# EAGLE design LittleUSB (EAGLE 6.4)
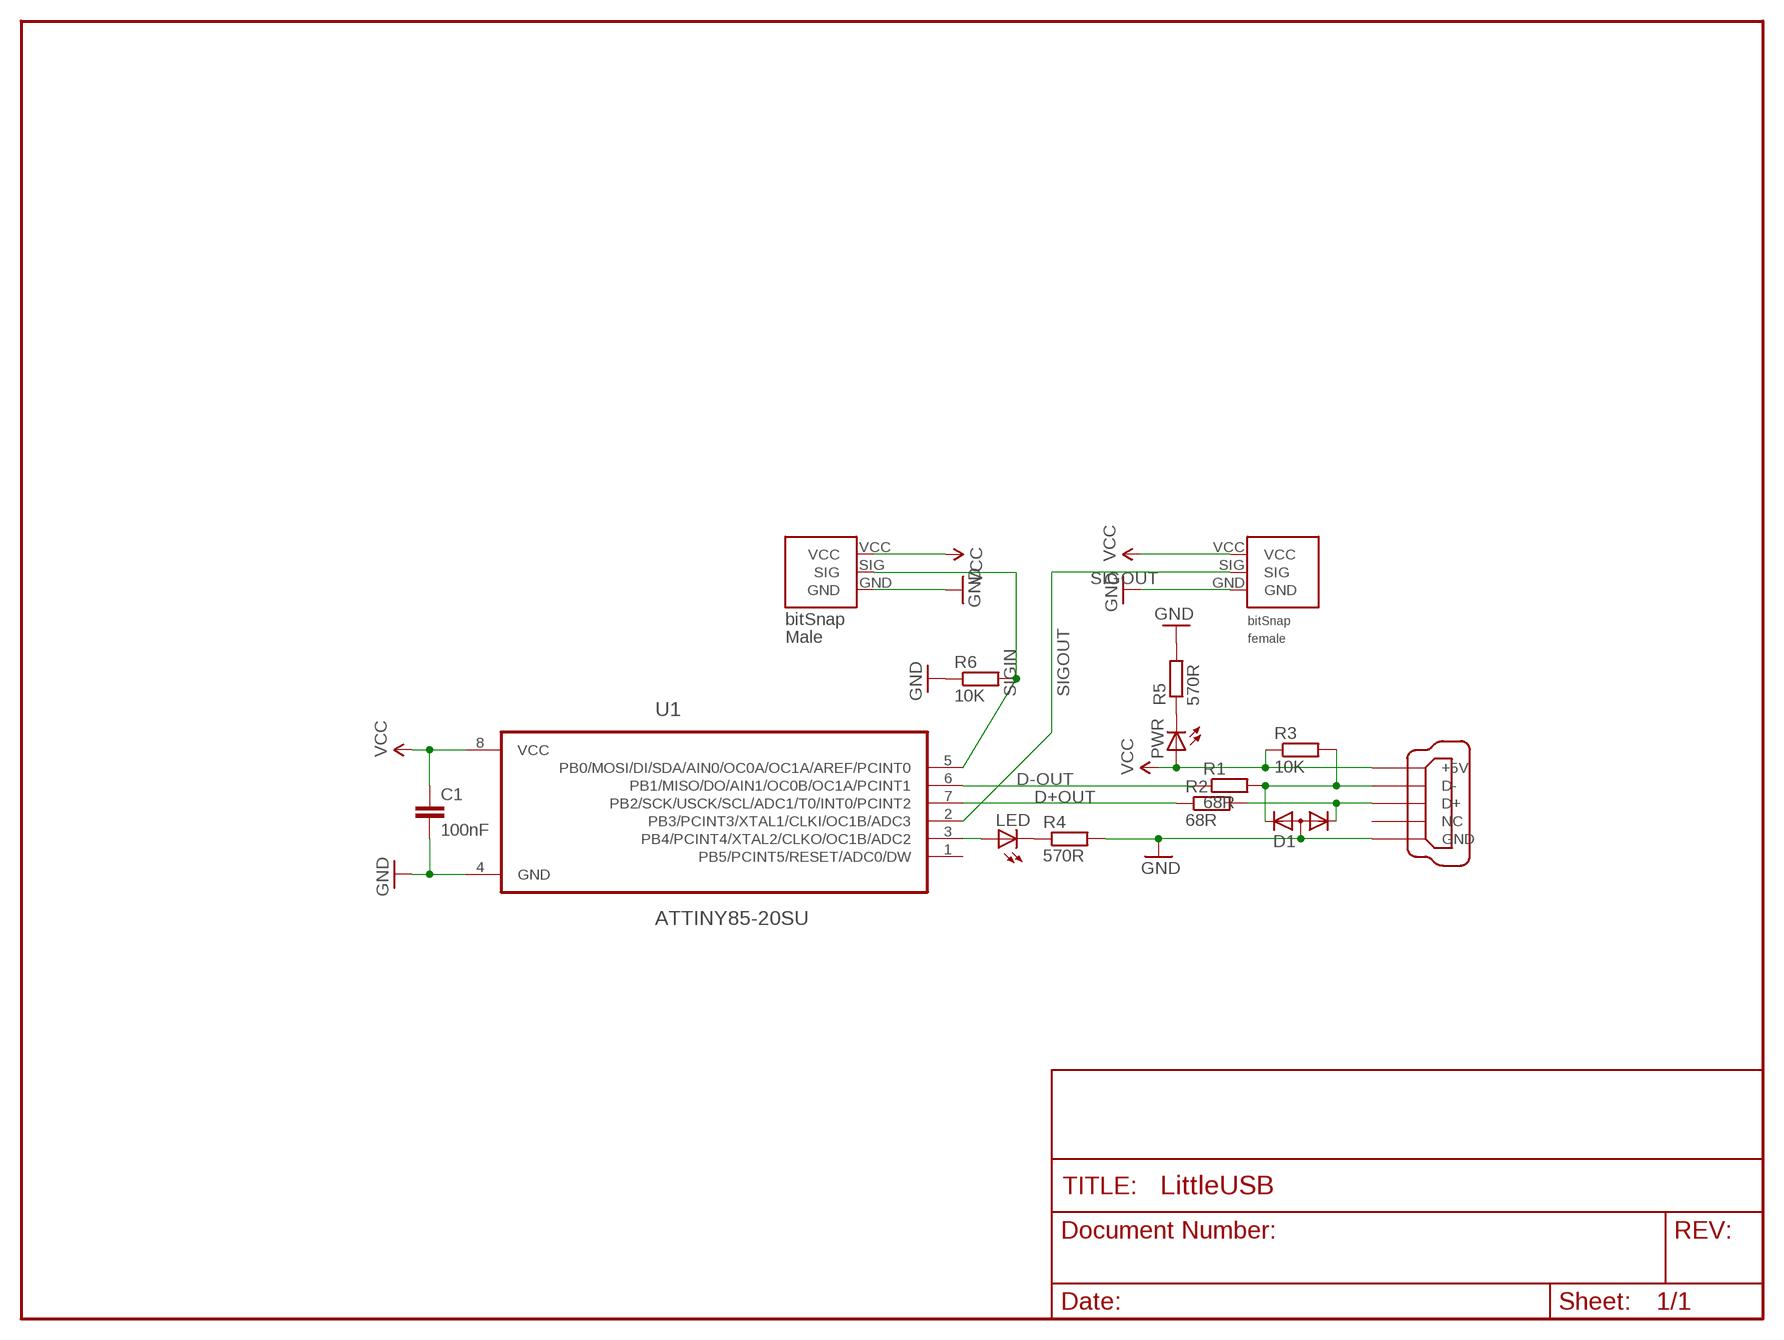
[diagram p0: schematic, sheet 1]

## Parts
C1  100nF  C-EUC0603  [C0603]
D1  DIODE-2CA|ACSOT23  [SOT23]
I3BSF  LITTLEBIT_FEMALE  [LITTLEBIT_FEMALE]
I3BSM  LITTLEBIT_MALE  [LITTLEBIT_MALE]
LED  LEDCHIPLED_0603  [CHIPLED_0603]
PWR  LEDCHIPLED_0603  [CHIPLED_0603]
R1  68R  R-EU_R0603  [R0603]
R2  68R  R-EU_R0603  [R0603]
R3  10K  R-EU_R0603  [R0603]
R4  570R  R-EU_R0603  [R0603]
R5  570R  R-EU_R0603  [R0603]
R6  10K  R-EU_R0603  [R0603]
U1  ATTINY85-20SU  [SOIC127P798X216-8N]
X1  MINI-USB-32005-301  [32005-301]

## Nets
D+OUT: R2.1 U1.7(PB2/SCK/USCK/SCL/ADC1/T0/INT0/PCINT2)
D-OUT: R1.1 U1.6(PB1/MISO/DO/AIN1/OC0B/OC1A/PCINT1)
GND: C1.2 D1.3(A) I3BSF.GND I3BSM.GND R4.2 R5.2 R6.1 U1.4(GND) X1.GND
N$1: LED.A U1.3(PB4/PCINT4/XTAL2/CLKO/OC1B/ADC2)
N$2: D1.2(K2) R1.2 R3.2 X1.D-
N$3: D1.1(K1) R2.2 X1.D+
N$4: LED.C R4.1
N$6: PWR.C R5.1
SIGIN: I3BSM.SIG R6.2 U1.5(PB0/MOSI/DI/SDA/AIN0/OC0A/OC1A/AREF/PCINT0)
SIGOUT: I3BSF.SIG U1.2(PB3/PCINT3/XTAL1/CLKI/OC1B/ADC3)
VCC: C1.1 I3BSF.VCC I3BSM.VCC PWR.A R3.1 U1.8(VCC) X1.+5V
Unconnected: U1.1(PB5/PCINT5/RESET/ADC0/DW) X1.NC

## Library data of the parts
C1 = rcl:C-EU: CAPACITOR, European symbol
D1 = diode:DIODE-2CA|AC: Dual DIODE Cathode-Anode|Anode-Cathode
I3BSF = MikesParts:LITTLEBIT_FEMALE
I3BSM = MikesParts:LITTLEBIT_MALE
LED PWR = led:LED: LED
R1-R6 = rcl:R-EU_: RESISTOR, European symbol
U1 = MikesParts:ATTINY85-20SU: 8-bit Microcontroller with In-System Programmable Flash; MPN: ATTINY85-20SU; OC_FARNELL: 1455164; OC_NEWARK: 58M3797; PACKAGE: SOIC-8; SUPPLIER: Atmel
X1 = MikesParts:MINI-USB-: MINI USB-B Conector Source: www.cypressindustries.com; OC_FARNELL: unknown; OC_NEWARK: unknown

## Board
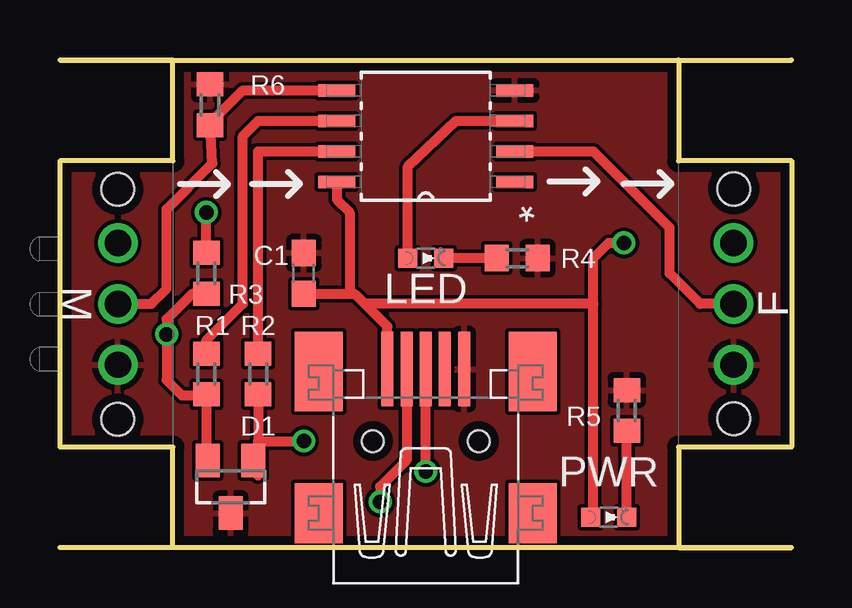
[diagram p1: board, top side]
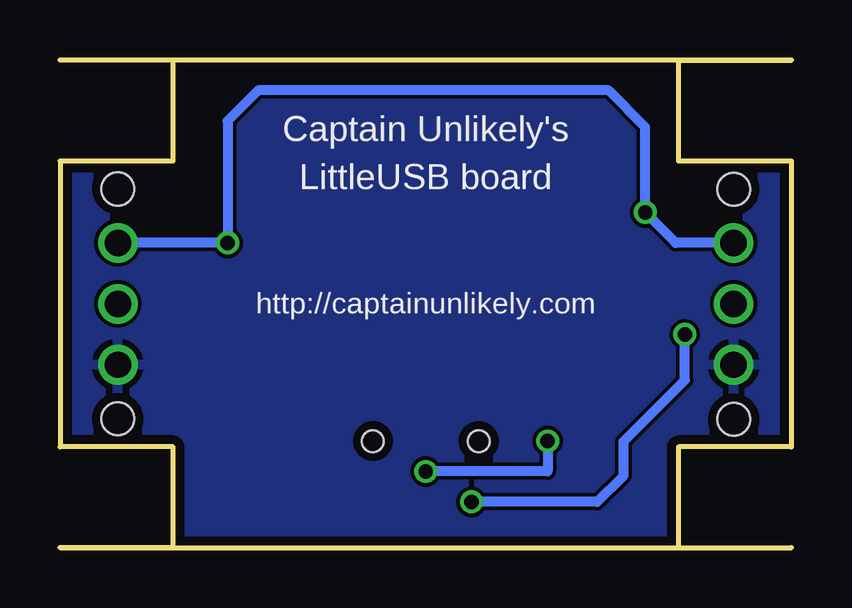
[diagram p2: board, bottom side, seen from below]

Size 30.48 x 20.32 mm. Coordinates in mm from the lower left corner, seen from the top.
Outline: 0,20.32 30.48,20.32
Outline: 30.48,0 0,0
Copper layers (1*16): Top 0.0356mm / dielectric 1.5011mm / Bottom 0.0356mm
Design rules "LaenPCBOrder": minimum track width 6mil, minimum drill 13mil, track to track 6mil, track to pad 6mil, pad to pad 6mil, via to via 6mil, smd to smd 6mil, copper to edge 15mil, drill to drill 6mil, minimum pad ring 7mil, minimum via ring 7mil, stop-mask expansion 4mil, vias tented up to drill 0mil, thermal gap 10mil

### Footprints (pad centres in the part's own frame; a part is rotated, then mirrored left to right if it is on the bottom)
C0603 = smd 1.1 x 1: 1 -0.85,0; 2 0.85,0
SOT23 = smd 1 x 1.4: 1 -0.95,-1.1; 2 0.95,-1.1; 3 0,1.1
LITTLEBIT_FEMALE = drill 1.1: GND 7.62,2.41; SIG 10.16,2.41; VCC 12.7,2.41 | hole 1.37: 14.95,2.41; 5.37,2.41
LITTLEBIT_MALE = drill 1.1: GND 12.7,2.41; SIG 10.16,2.41; VCC 7.62,2.41 | hole 1.37: 14.965,2.41; 5.385,2.41
CHIPLED_0603 = smd 0.8 x 0.8: A 0,-0.75; C 0,0.75
R0603 = smd 1 x 1.1: 1 -0.85,0; 2 0.85,0
SOIC127P798X216-8N = smd 1.549 x 0.533: 1 -3.708,1.905; 2 -3.708,0.635; 3 -3.708,-0.635; 4 -3.708,-1.905; 5 3.708,-1.905; 6 3.708,-0.635; 7 3.708,0.635; 8 3.708,1.905
32005-301 = smd 3.1 x 0.5: +5V 3,1.6; D+ 3,0; D- 3,0.8; GND 3,-1.6; NC 3,-0.8 | smd 2.5 x 2: M1 -3,-4.45; M2 -3,4.45 | smd 3.3 x 2: M3 2.9,4.45; M4 2.9,-4.45 | hole 0.9: 0,2.2; 0,-2.2

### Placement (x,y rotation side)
C1  10.16,11.43 90 top
D1  7.11,2.54 180 top
I3BSF  30.48,0 90 top
I3BSM  0,20.32 270 top
LED  15.24,12.06 270 top
PWR  22.86,1.27 270 top
R1  6.1,7.24 270 top
R2  8.26,7.24 270 top
R3  6.1,11.43 270 top
R4  19.05,12.06 0 top
R5  23.62,5.71 90 top
R6  6.25,18.45 270 top
U1  15.24,17.14 180 top
X1  15.24,4.45 90 top

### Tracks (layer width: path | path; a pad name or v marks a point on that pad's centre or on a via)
D+OUT
  Top 0.406: U1.7 8.26,16.51 R2.1
D-OUT
  Top 0.406: R1.1 6.1,8.64 7.62,10.16 7.62,17.14 8.26,17.78 U1.6
GND
  pour Top: 0,0 0,20.32 30.48,20.32 30.48,0
  pour Bottom: 0,0 0,20.32 30.48,20.32 30.48,0
N$1
  Top 0.406: LED.A 14.49,15.88 16.51,17.78 U1.3
N$2  (via drill 0.6)
  Top 0.406: X1.D- 14.44,3.65 13.34,2.54 v13.34,1.91 | R3.2 5.5,10.58 4.45,9.53 v4.45,8.89 4.45,6.99 5.08,6.35 6.06,6.35 R1.2 6.1,3.71 D1.2
  Bottom 0.406: v13.34,1.91 8.1,1.91 7,3 7,4.43 4.45,6.99 v4.45,8.89
N$3  (via drill 0.6)
  Top 0.406: D1.1 8.26,3 8.26,4.45 | R2.2 8.26,4.45 | 8.26,4.45 v10.16,4.45 | v15.24,3.17 X1.D+
  Bottom 0.406: v10.16,4.45 10.16,3.17 v15.24,3.17
N$4
  Top 0.406: R4.1 LED.C
N$6
  Top 0.406: PWR.C 23.62,2.85 R5.1
SIGIN
  Top 0.406: I3BSM.SIG 3.81,10.16 4.45,10.79 4.45,14.11 6.35,16.01 R6.2 6.35,17.78 7.62,19.05 U1.5
SIGOUT
  Top 0.406: I3BSF.SIG 26.67,10.16 25.4,11.43 25.4,13.34 22.23,16.51 U1.2
VCC  (via drill 0.6)
  Top 0.406: C1.1 12.06,10.58 | 12.06,10.58 12.28,10.58 12.7,10.16 | 12.7,10.16 13.64,9.22 X1.+5V | R3.1 v6.1,13.97 | U1.8 11.53,14.5 12.06,13.97 12.06,10.58 | 22.23,10.16 22.23,1.39 PWR.A | 22.23,10.16 12.7,10.16 | 22.23,10.16 22.23,12.06 22.86,12.7 v23.5,12.7
  Bottom 0.406: I3BSF.VCC v23.5,12.7 23.5,17.78 22.23,19.05 7.62,19.05 6.1,17.53 v6.1,13.97 4.83,12.7 I3BSM.VCC

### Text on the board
bNames: Captain Unlikely's | LittleUSB board | http://captainunlikely.com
